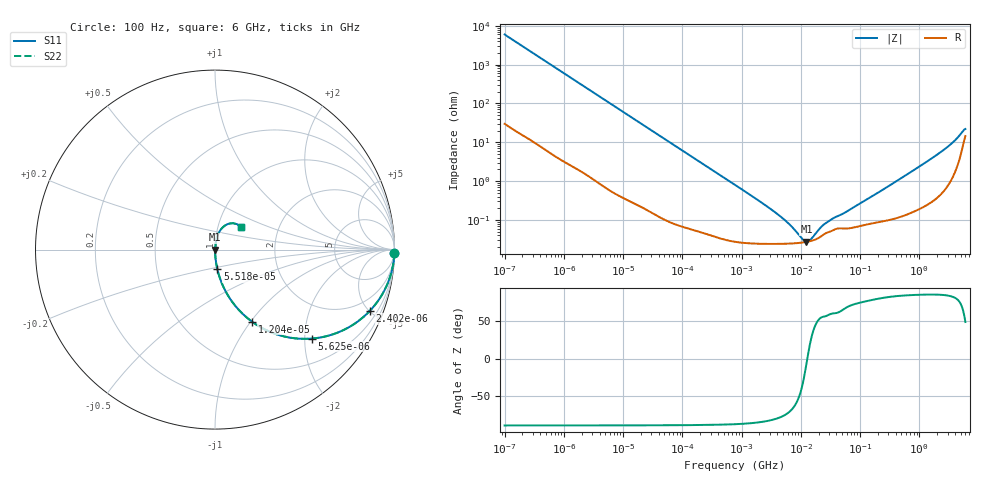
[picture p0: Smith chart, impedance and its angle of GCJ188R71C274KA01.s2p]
!Murata Part Number: GCJ188R71C274KA01
!These Parameters are Measured in Series Mode Connection
!Data Generated on Mar 13, 2026
!  o--ll--o
!Port1  Port2
!  o------o
!Operation Temp=25[degC], DC Bias Voltage=0[V]
!Freq. Start=100[Hz] Stop=6[GHz] 401[Steps]
# Hz S RI R 50
!Freq.(Hz) S11(Real) S11(Imag) S21(Real) S21(Imag) S12(Real) S12(Imag) S22(Real) S22(Imag)
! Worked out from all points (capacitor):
!   401 points, 100 Hz to 6 GHz, reference 50 ohm
!   read as one part in series: C = 265 nF near 109 Hz
!   lowest |Z| = 27.2 mohm at 12.44 MHz (marker M1)
!   series resonance near 12.89 MHz, so ESL is about 570 pH
!   S11 on the Smith chart (normalised r, x): 100 Hz: open; 2.402 kHz: 1.03, -5.04; 5.625 kHz: 1.01, -2.16; 12.04 kHz: 1.01, -1.01; 55.18 kHz: 1.00, -0.22; 6 GHz: 1.29, +0.33
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100  0.9996 -0.0167  0.000361 0.0167  0.000361 0.0167  0.9996 -0.0167
600  0.9897 -0.0983  0.0103 0.0983  0.0103 0.0983  0.9897 -0.0983
2008  0.8995 -0.2978  0.1005 0.2978  0.1005 0.2978  0.8995 -0.2978
2402  0.8628 -0.3412  0.1372 0.3412  0.1372 0.3412  0.8628 -0.3412
5625  0.5385 -0.4957  0.4615 0.4957  0.4615 0.4957  0.5385 -0.4957
12041  0.2053 -0.4008  0.7947 0.4008  0.7947 0.4008  0.2053 -0.4008
20606  0.0823 -0.2713  0.9177 0.2713  0.9177 0.2713  0.0823 -0.2713
40335  0.0236 -0.148  0.9764 0.148  0.9764 0.148  0.0236 -0.148
55182  0.0131 -0.1095  0.9869 0.1095  0.9869 0.1095  0.0131 -0.1095
161617  0.00198 -0.038  0.998 0.038  0.998 0.038  0.00198 -0.038
774597  0.000336 -0.00799  0.9997 0.00799  0.9997 0.00799  0.000336 -0.00799
4246196  0.000243 -0.00131  0.9998 0.00131  0.9998 0.00131  0.000243 -0.00131
6644369  0.000246 -0.000688  0.9998 0.000688  0.9998 0.000688  0.000246 -0.000688
1.087309e7  0.000262 -0.000166  0.9997 0.000166  0.9997 0.000166  0.000262 -0.000166
1.243624e7  0.00027 -3.48e-05  0.9997 3.48e-05  0.9997 3.48e-05  0.00027 -3.48e-05
1.555665e7  0.000292 0.000183  0.9997 -0.000183  0.9997 -0.000183  0.000292 0.000183
2.662322e7  0.000456 0.000697  0.9995 -0.000697  0.9995 -0.000697  0.000456 0.000697
3.124326e8  0.00105 0.00755  0.9989 -0.00755  0.9989 -0.00755  0.00105 0.00755
1.565993e9  0.00413 0.0368  0.9959 -0.0368  0.9959 -0.0368  0.00413 0.0368
3.352442e9  0.0169 0.0846  0.9831 -0.0846  0.9831 -0.0846  0.0169 0.0846
4.586474e9  0.0458 0.1265  0.9542 -0.1265  0.9542 -0.1265  0.0458 0.1265
6e9  0.1441 0.1239  0.8559 -0.1239  0.8559 -0.1239  0.1441 0.1239
